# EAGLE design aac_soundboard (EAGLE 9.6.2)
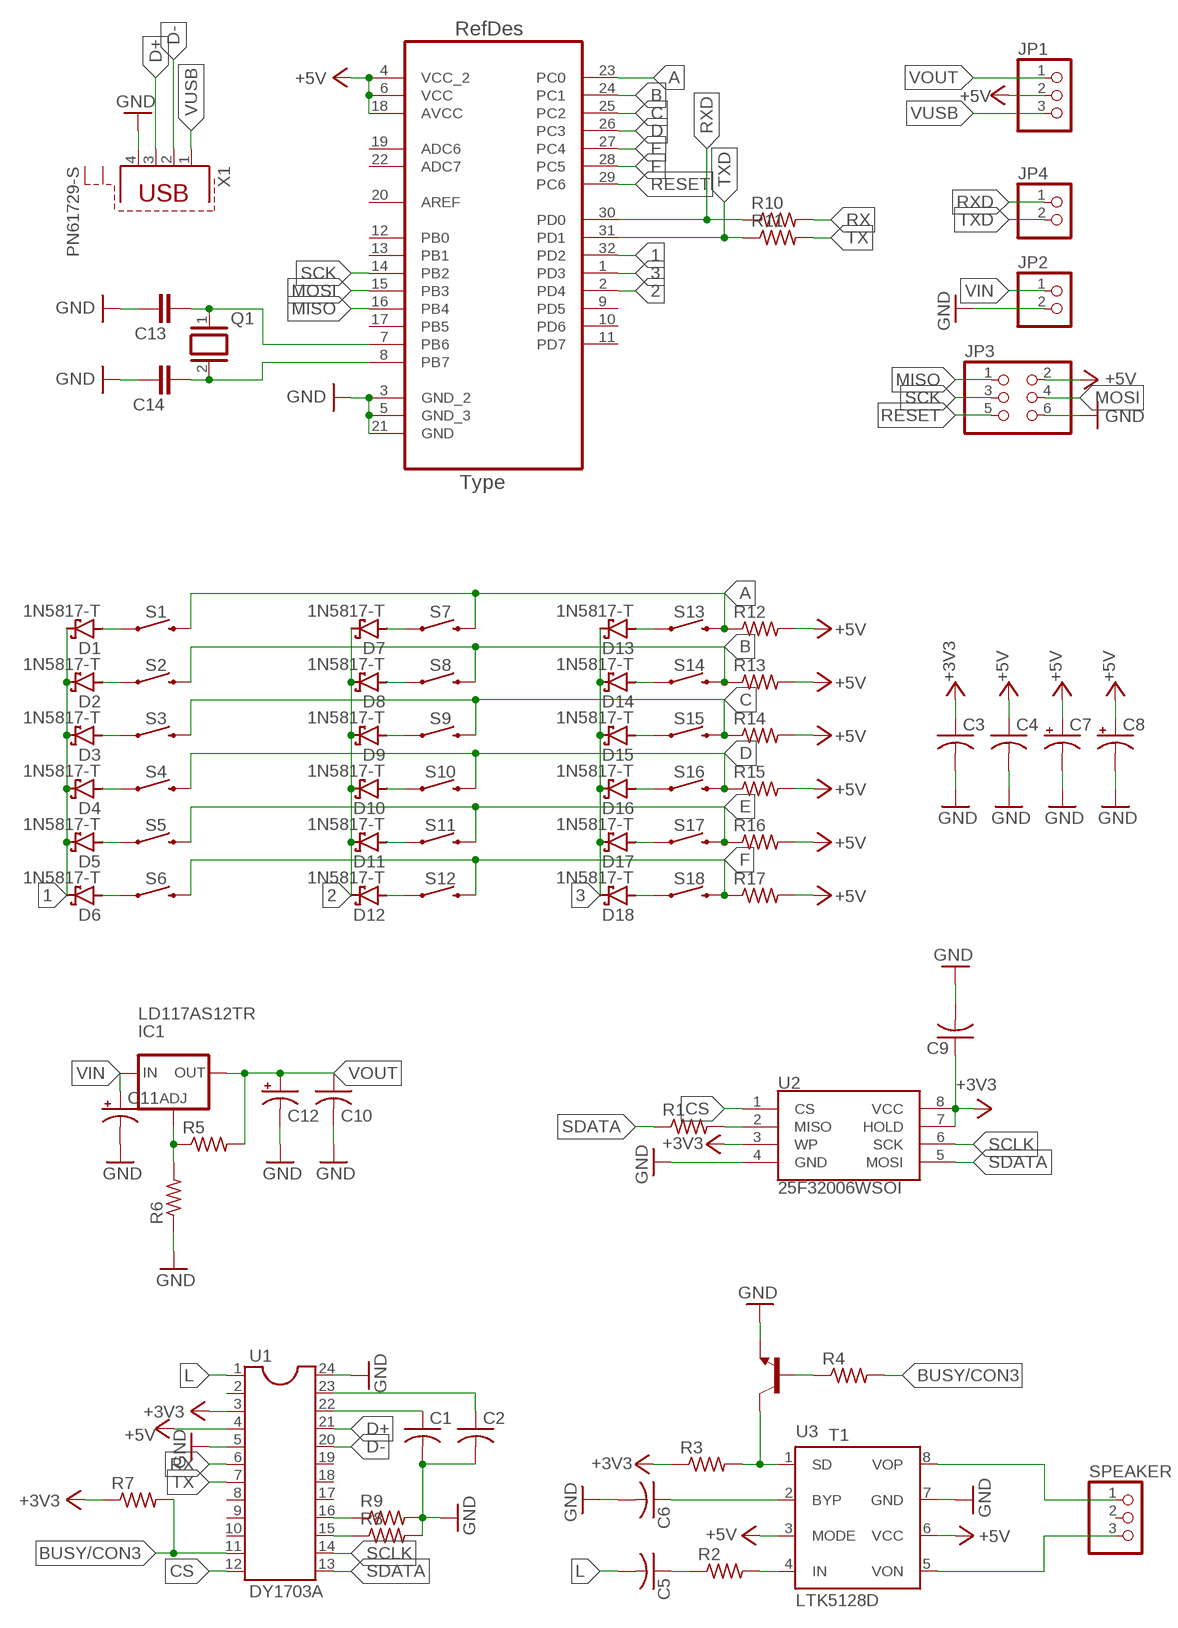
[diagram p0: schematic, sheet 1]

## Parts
ATMEGA328  ATMEGA328P-AU  [QFP80P900X900X120-32N]
C1  C-US050-025X075  [C050-025X075]
C2  C-US050-025X075  [C050-025X075]
C3  C-US050-025X075  [C050-025X075]
C4  C-US050-025X075  [C050-025X075]
C5  C-US050-025X075  [C050-025X075]
C6  C-US050-025X075  [C050-025X075]
C7  CPOL-USE2.5-6  [E2,5-6]
C8  CPOL-USE2.5-6  [E2,5-6]
C9  C-US050-025X075  [C050-025X075]
C10  C-US050-025X075  [C050-025X075]
C11  CPOL-USE2.5-6  [E2,5-6]
C12  CPOL-USE2.5-6  [E2,5-6]
C13  C-EU025-024X044  [C025-024X044]
C14  C-EU025-024X044  [C025-024X044]
D1  1N5817-T  [DO41-7.6]
D2  1N5817-T  [DO41-7.6]
D3  1N5817-T  [DO41-7.6]
D4  1N5817-T  [DO41-7.6]
D5  1N5817-T  [DO41-7.6]
D6  1N5817-T  [DO41-7.6]
D7  1N5817-T  [DO41-7.6]
D8  1N5817-T  [DO41-7.6]
D9  1N5817-T  [DO41-7.6]
D10  1N5817-T  [DO41-7.6]
D11  1N5817-T  [DO41-7.6]
D12  1N5817-T  [DO41-7.6]
D13  1N5817-T  [DO41-7.6]
D14  1N5817-T  [DO41-7.6]
D15  1N5817-T  [DO41-7.6]
D16  1N5817-T  [DO41-7.6]
D17  1N5817-T  [DO41-7.6]
D18  1N5817-T  [DO41-7.6]
IC1  LD117AS12TR  [SOT223]
JP1  PINHD-1X3  [1X03]
JP2  PINHD-1X2  [1X02]
JP3  PINHD-2X3  [2X03]
JP4  PINHD-1X2  [1X02]
Q1  XTAL/S  [QS]
R1  R-US_0204/7  [0204/7]
R2  R-US_0204/7  [0204/7]
R3  R-US_0204/7  [0204/7]
R4  R-US_0204/7  [0204/7]
R5  R-US_0204/7  [0204/7]
R6  R-US_0204/7  [0204/7]
R7  R-US_0204/7  [0204/7]
R8  R-US_0204/7  [0204/7]
R9  R-US_0204/7  [0204/7]
R10  R-US_0204/7  [0204/7]
R11  R-US_0204/7  [0204/7]
R12  R-US_0204/7  [0204/7]
R13  R-US_0204/7  [0204/7]
R14  R-US_0204/7  [0204/7]
R15  R-US_0204/7  [0204/7]
R16  R-US_0204/7  [0204/7]
R17  R-US_0204/7  [0204/7]
S1  MOMENTARY-SWITCH-SPST-PTH-12MM  [TACTILE_SWITCH_PTH_12MM]
S2  MOMENTARY-SWITCH-SPST-PTH-12MM  [TACTILE_SWITCH_PTH_12MM]
S3  MOMENTARY-SWITCH-SPST-PTH-12MM  [TACTILE_SWITCH_PTH_12MM]
S4  MOMENTARY-SWITCH-SPST-PTH-12MM  [TACTILE_SWITCH_PTH_12MM]
S5  MOMENTARY-SWITCH-SPST-PTH-12MM  [TACTILE_SWITCH_PTH_12MM]
S6  MOMENTARY-SWITCH-SPST-PTH-12MM  [TACTILE_SWITCH_PTH_12MM]
S7  MOMENTARY-SWITCH-SPST-PTH-12MM  [TACTILE_SWITCH_PTH_12MM]
S8  MOMENTARY-SWITCH-SPST-PTH-12MM  [TACTILE_SWITCH_PTH_12MM]
S9  MOMENTARY-SWITCH-SPST-PTH-12MM  [TACTILE_SWITCH_PTH_12MM]
S10  MOMENTARY-SWITCH-SPST-PTH-12MM  [TACTILE_SWITCH_PTH_12MM]
S11  MOMENTARY-SWITCH-SPST-PTH-12MM  [TACTILE_SWITCH_PTH_12MM]
S12  MOMENTARY-SWITCH-SPST-PTH-12MM  [TACTILE_SWITCH_PTH_12MM]
S13  MOMENTARY-SWITCH-SPST-PTH-12MM  [TACTILE_SWITCH_PTH_12MM]
S14  MOMENTARY-SWITCH-SPST-PTH-12MM  [TACTILE_SWITCH_PTH_12MM]
S15  MOMENTARY-SWITCH-SPST-PTH-12MM  [TACTILE_SWITCH_PTH_12MM]
S16  MOMENTARY-SWITCH-SPST-PTH-12MM  [TACTILE_SWITCH_PTH_12MM]
S17  MOMENTARY-SWITCH-SPST-PTH-12MM  [TACTILE_SWITCH_PTH_12MM]
S18  MOMENTARY-SWITCH-SPST-PTH-12MM  [TACTILE_SWITCH_PTH_12MM]
SPEAKER  PINHD-1X3  [1X03]
T1  -NPN-TO92-EBC  [TO92-EBC]
U1  DY1703A  [TSSOP24]
U2  25F32006WSOI  SPI_FLASH-X25XXSMD1  [SO08-EIAJ]
U3  LTK5128D  [SO08_PAD]
X1  PN61729-S  [PN61729-S]

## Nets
1: ATMEGA328.32(PD2) D1.C D2.C D3.C D4.C D5.C D6.C
2: ATMEGA328.2(PD4) D7.C D8.C D9.C D10.C D11.C D12.C
3: ATMEGA328.1(PD3) D13.C D14.C D15.C D16.C D17.C D18.C
+3V3: C3.1 C9.1 R3.1 R7.1 U1.3 U2.3(WP) U2.7(HOLD) U2.8(VCC)
+5V: ATMEGA328.4(VCC_2) ATMEGA328.6(VCC) ATMEGA328.18(AVCC) C4.1 C7.+ C8.+ JP1.2 JP3.2 R12.2 R13.2 R14.2 R15.2 R16.2 R17.2 U1.4 U3.3(MODE) U3.6(VCC)
A: ATMEGA328.23(PC0) R12.1 S1.3 S7.3 S13.3
B: ATMEGA328.24(PC1) R13.1 S2.3 S8.3 S14.3
BUSY/CON3: R4.2 R7.2 U1.11
C: ATMEGA328.25(PC2) R14.1 S3.3 S9.3 S15.3
CON1: R9.1 U1.16
CON2: R8.1 U1.15
CS: U1.12 U2.1(CS)
D: ATMEGA328.26(PC3) R15.1 S4.3 S10.3 S16.3
D+: U1.21 X1.3
D-: U1.20 X1.2
E: ATMEGA328.27(PC4) R16.1 S5.3 S11.3 S17.3
F: ATMEGA328.28(PC5) R17.1 S6.3 S12.3 S18.3
GND: ATMEGA328.3(GND_2) ATMEGA328.5(GND_3) ATMEGA328.21(GND) C1.2 C2.2 C3.2 C4.2 C6.2 C7.- C8.- C9.2 C10.2 C11.- C12.- C13.2 C14.2 JP2.2 JP3.6 R6.1 R8.2 R9.2 T1.E U1.5 U1.24 U2.4(GND) U3.7(GND) X1.4
L: C5.2 U1.1
MISO: ATMEGA328.16(PB4) JP3.1
MOSI: ATMEGA328.15(PB3) JP3.4
N$1: D1.A S1.1
N$2: D2.A S2.1
N$3: D3.A S3.1
N$4: D4.A S4.1
N$5: D5.A S5.1
N$6: D6.A S6.1
N$7: D7.A S7.1
N$8: D8.A S8.1
N$9: D9.A S9.1
N$10: D10.A S10.1
N$11: D11.A S11.1
N$12: D12.A S12.1
N$13: D13.A S13.1
N$14: D14.A S14.1
N$15: D15.A S15.1
N$16: D16.A S16.1
N$17: D17.A S17.1
N$18: D18.A S18.1
N$28: R1.2 U2.2(MISO)
N$29: R2.2 U3.4(IN)
N$30: C6.1 U3.2(BYP)
N$31: C5.1 R2.1
N$32: R3.2 T1.C U3.1(SD)
N$33: R4.1 T1.B
N$34: C1.1 U1.22
N$35: C2.1 U1.23
N$36: IC1.1(ADJ) R5.1 R6.2
N$37: SPEAKER.1 U3.8(VOP)
N$38: SPEAKER.3 U3.5(VON)
N$40: ATMEGA328.8(PB7) C14.1 Q1.2
N$41: ATMEGA328.7(PB6) C13.1 Q1.1
RESET: ATMEGA328.29(PC6) JP3.5
RX: R10.2 U1.6
RXD: ATMEGA328.30(PD0) JP4.1 R10.1
SCK: ATMEGA328.14(PB2) JP3.3
SCLK: U1.14 U2.6(SCK)
SDATA: R1.1 U1.13 U2.5(MOSI)
TX: R11.2 U1.7
TXD: ATMEGA328.31(PD1) JP4.2 R11.1
VIN: C11.+ IC1.3(IN) JP2.1
VOUT: C10.1 C12.+ IC1.4(OUT) JP1.1 R5.2
VUSB: JP1.3 X1.1
Unconnected: ATMEGA328.9(PD5) ATMEGA328.10(PD6) ATMEGA328.11(PD7) ATMEGA328.12(PB0) ATMEGA328.13(PB1) ATMEGA328.17(PB5) ATMEGA328.19(ADC6) ATMEGA328.20(AREF) ATMEGA328.22(ADC7) SPEAKER.2 U1.2 U1.8 U1.9 U1.10 U1.17 U1.18 U1.19 X1.S1 X1.S2

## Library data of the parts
ATMEGA328 = Atmel-ATMEGA328P-AU:ATMEGA328P-AU; DESCRIPTION: 8-bit Microcontroller with In-System Programmable Flash; MPN: ATMEGA328P-AU; OC_FARNELL: 1715486; OC_NEWARK: 14R4631; PACKAGE: TQFP-32; SUPPLIER: Atmel
C1-C6 C9 C10 = rcl:C-US: CAPACITOR, American symbol; SPICEPREFIX: C
C7 C8 C11 C12 = rcl:CPOL-US: POLARIZED CAPACITOR, American symbol; SPICEPREFIX: C
C13 C14 = rcl:C-EU: CAPACITOR, European symbol; SPICEPREFIX: C
D1-D18 = diode:1N581*: 1.0A SCHOTTKY BARRIER RECTIFIER
IC1 = v-reg:LD117A?*: Low drop fixed and adjustable positive voltage regulators 1 A Source: http://www.st.com/stonline/products/literature/ds/7194/ld1117axx.pdf
JP1 SPEAKER = pinhead:PINHD-1X3: PIN HEADER
JP2 JP4 = pinhead:PINHD-1X2: PIN HEADER
JP3 = pinhead:PINHD-2X3: PIN HEADER
Q1 = special:XTAL/S: CRYSTAL
R1-R17 = rcl:R-US_: RESISTOR, American symbol; SPICEPREFIX: R
S1-S18 = SparkFun-Switches:MOMENTARY-SWITCH-SPST: Momentary Switch (Pushbutton) - SPST; PROD_ID: SWCH-09185; SF_SKU: COM-09190
T1 = transistor:*-NPN-: NPN Transistror BF959 corrected 2008.03.06
U1 = smd_sop8_amp:DY1703A
U2 = SparkFun-IC-Memory:SPI_FLASH-X25XX: 32M Serial Flash Memory 8pin SPI Flash series x25xx. Works with devices like W25X32 and BR25L32 Datasheet SparkFun Products SparkFun Venus GPS Logger (GPS-10920); PROD_ID: IC-09109
U3 = smd_sop8_amp:LTK5128D
X1 = con-berg:PN61729-S: BERG USB connector; OC_FARNELL: unknown; OC_NEWARK: unknown

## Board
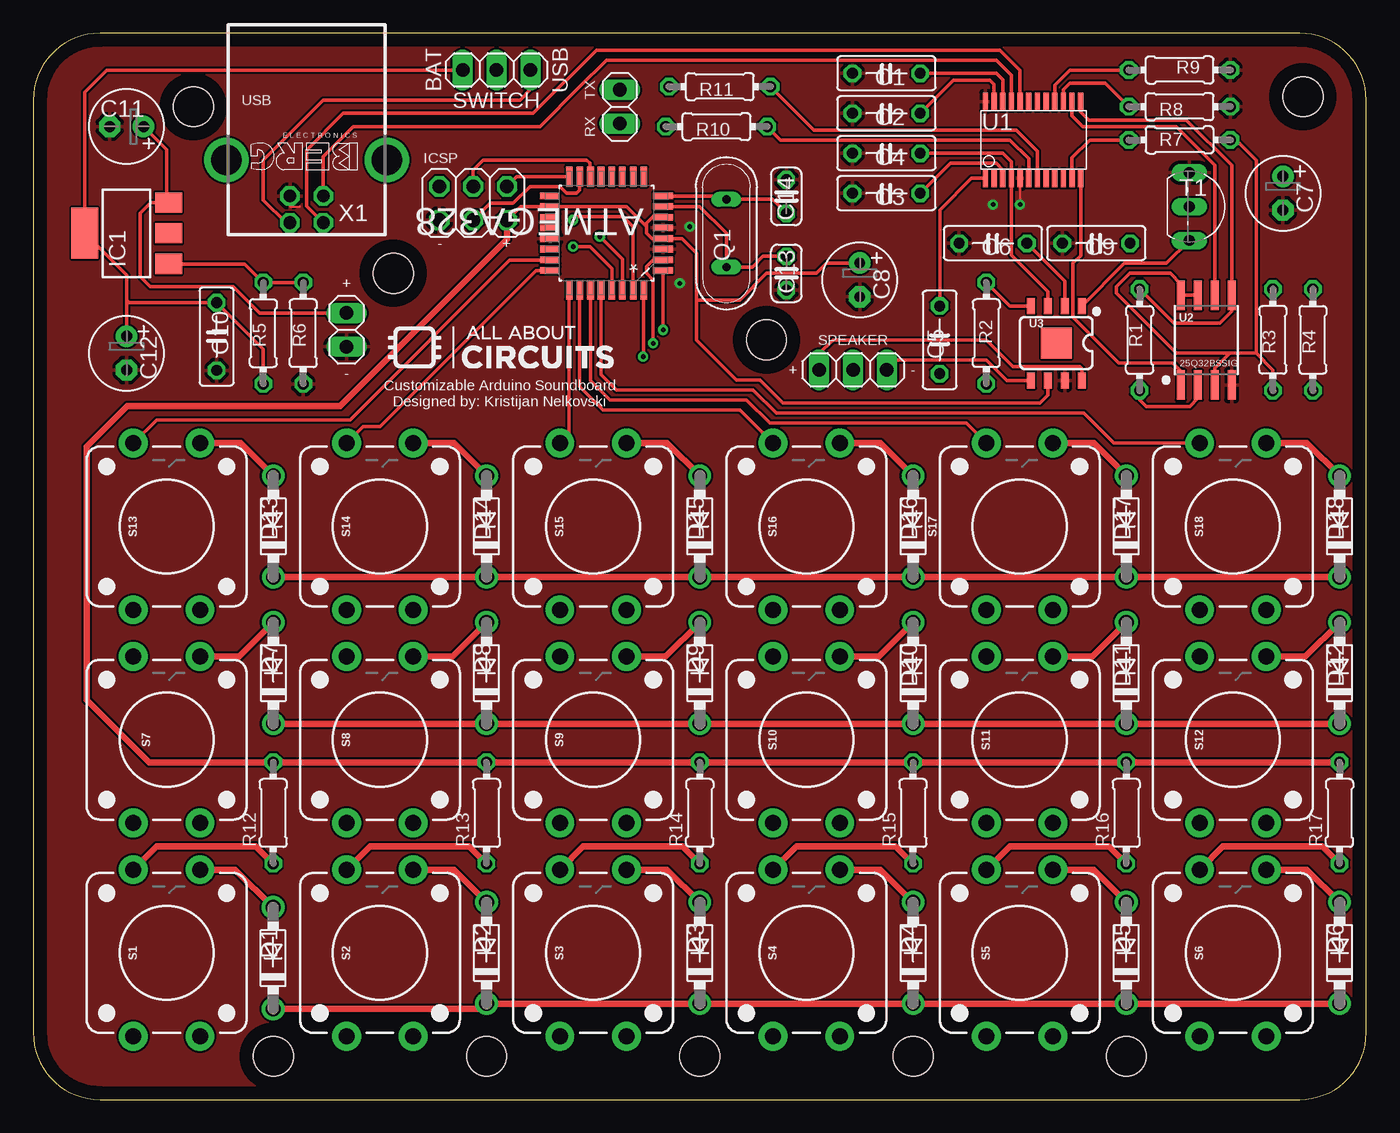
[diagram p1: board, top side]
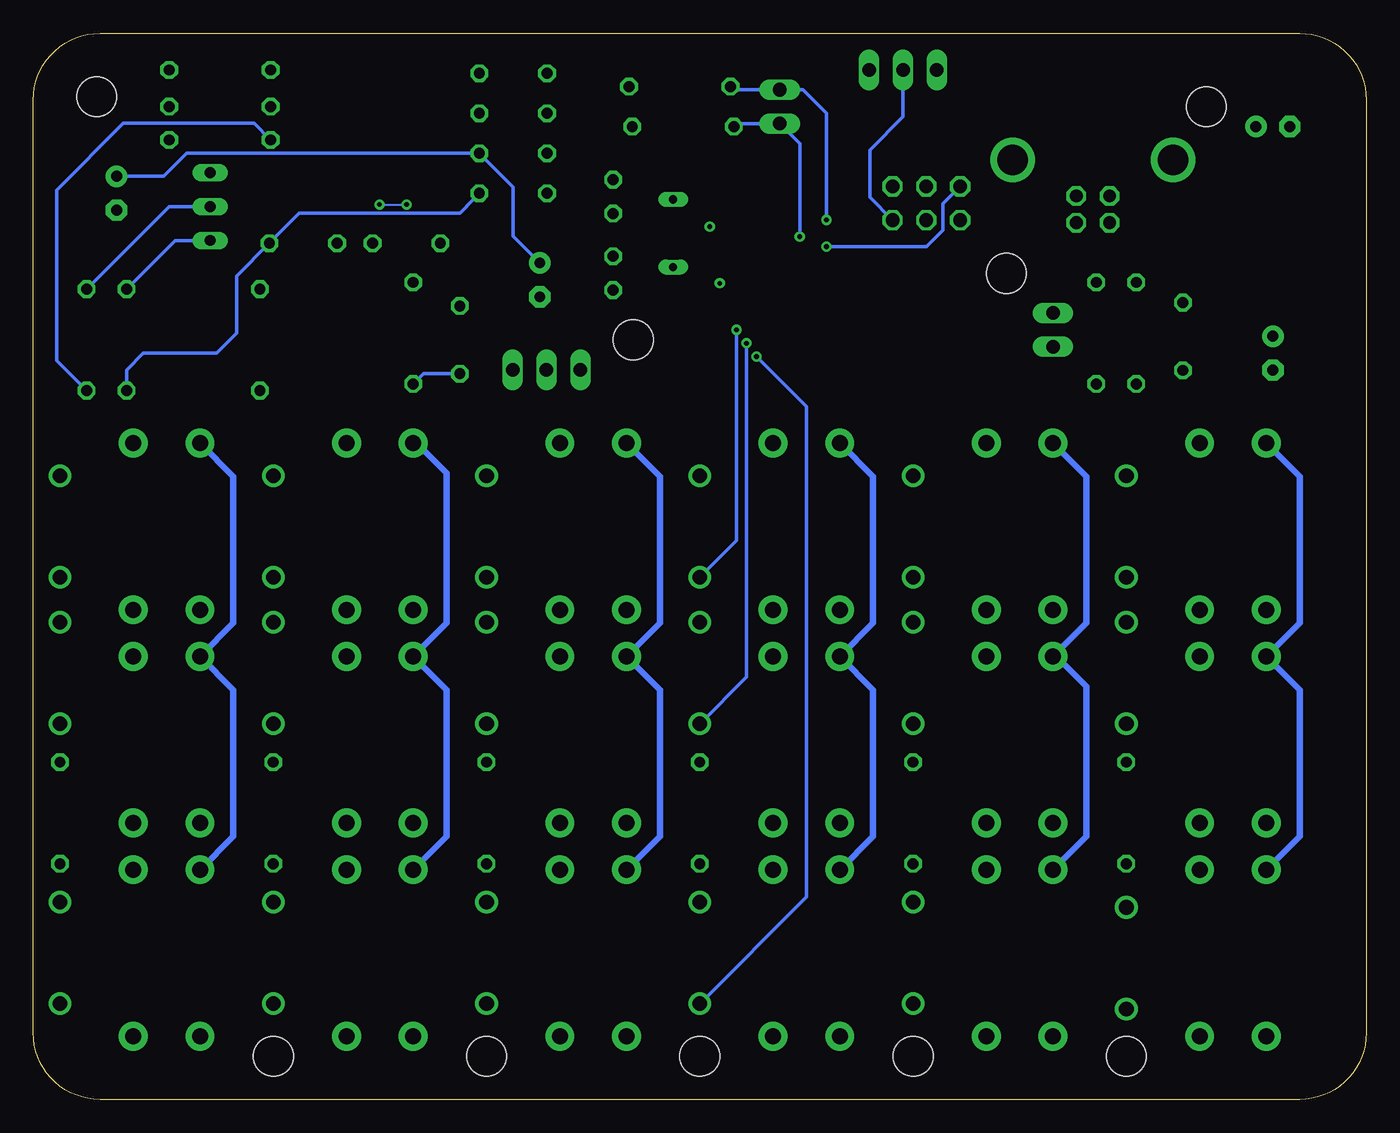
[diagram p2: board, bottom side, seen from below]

Size 100 x 80 mm. Coordinates in mm from the lower left corner, seen from the top.
Outline: 0,75 0,5 arc90 5,0 95,0 arc90 100,5 100,75 arc90 95,80 5,80 arc90 0,75
Copper layers (1*16): Top 0.035mm / dielectric 1.5mm / Bottom 0.035mm
Design rules "default": minimum track width 6mil, minimum drill 0.35mm, track to track 6mil, track to pad 6mil, pad to pad 6mil, via to via 6mil, smd to smd 6mil, copper to edge 40mil, drill to drill 6mil, minimum pad ring 10mil, minimum via ring 8mil, stop-mask expansion 4mil, vias tented up to drill 0mil, thermal gap 10mil
Holes 3 mm at 18,3.25 34,3.25 50,3.25 66,3.25 82,3.25 55,57 27,62 12,74.5 95.25,75.25

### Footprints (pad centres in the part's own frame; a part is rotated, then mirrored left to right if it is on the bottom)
QFP80P900X900X120-32N = smd 1.473 x 0.508: 1 -4.242,2.794; 2 -4.242,2.007; 3 -4.242,1.194; 4 -4.242,0.406; 5 -4.242,-0.406; 6 -4.242,-1.194; 7 -4.242,-2.007; 8 -4.242,-2.794; 17 4.242,-2.794; 18 4.242,-2.007; 19 4.242,-1.194; 20 4.242,-0.406; 21 4.242,0.406; 22 4.242,1.194; 23 4.242,2.007; 24 4.242,2.794 | smd 0.508 x 1.473: 9 -2.794,-4.242; 10 -2.007,-4.242; 11 -1.194,-4.242; 12 -0.406,-4.242; 13 0.406,-4.242; 14 1.194,-4.242; 15 2.007,-4.242; 16 2.794,-4.242; 25 2.794,4.242; 26 2.007,4.242; 27 1.194,4.242; 28 0.406,4.242; 29 -0.406,4.242; 30 -1.194,4.242; 31 -2.007,4.242; 32 -2.794,4.242
C050-025X075 = drill 0.813 octagon: 1 -2.54,0; 2 2.54,0
E2,5-6 = drill 0.813 pad 1.6: + -1.27,0 | drill 0.813 pad 1.6 octagon: - 1.27,0
C025-024X044 = drill 0.813 octagon: 1 -1.27,0; 2 1.27,0
DO41-7.6 = drill 1.1 pad 1.7: A 3.81,0; C -3.81,0
SOT223 = smd 1.5 x 2: 1 -2.3,-3.15; 2 0,-3.15; 3 2.3,-3.15 | smd 3.8 x 2: 4 0,3.15
1X03 = drill 1.016 long: 1 -2.54,0; 2 0,0; 3 2.54,0
1X02 = drill 1.016 long: 1 -1.27,0; 2 1.27,0
2X03 = drill 1.016 octagon: 1 -2.54,-1.27; 2 -2.54,1.27; 3 0,-1.27; 4 0,1.27; 5 2.54,-1.27; 6 2.54,1.27
QS = drill 0.61 long: 1 -2.54,0; 2 2.54,0
0204/7 = drill 0.813 octagon: 1 -3.81,0; 2 3.81,0
TACTILE_SWITCH_PTH_12MM = drill 1.2 pad 2.159: 1 6.25,-2.5; 2 -6.25,-2.5; 3 6.25,2.5; 4 -6.25,2.5
TO92-EBC = drill 0.813 long: B 0,-1.27; C 2.54,-1.27; E -2.54,-1.27
TSSOP24 = smd 0.4 x 1.35: 1 -3.575,-2.875; 2 -2.925,-2.875; 3 -2.275,-2.875; 4 -1.625,-2.875; 5 -0.975,-2.875; 6 -0.325,-2.875; 7 0.325,-2.875; 8 0.975,-2.875; 9 1.625,-2.875; 10 2.275,-2.875; 11 2.93,-2.872; 12 3.58,-2.872; 13 3.573,2.875; 14 2.923,2.875; 15 2.275,2.875; 16 1.625,2.875; 17 0.975,2.875; 18 0.325,2.875; 19 -0.325,2.875; 20 -0.975,2.875; 21 -1.625,2.875; 22 -2.275,2.875; 23 -2.925,2.875; 24 -3.575,2.875
SO08-EIAJ = smd 0.61 x 2.21: 1 -1.905,-3.378; 2 -0.635,-3.378; 3 0.635,-3.378; 4 1.905,-3.378; 5 1.905,3.353; 6 0.635,3.353; 7 -0.635,3.353; 8 -1.905,3.353
SO08_PAD = smd 0.6 x 1.2: 1 -1.905,-2.8; 2 -0.635,-2.8; 3 0.635,-2.8; 4 1.905,-2.8; 5 1.905,2.8; 6 0.635,2.8; 7 -0.635,2.8; 8 -1.905,2.8 | smd 2.311 x 2.311: PAD 0,0
PN61729-S = drill 0.95 octagon: 1 1.25,4.71; 2 -1.25,4.71; 3 -1.25,2.71; 4 1.25,2.71 | drill 2.3 pad 2.9: S1 -6.02,0; S2 6.02,0

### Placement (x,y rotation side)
ATMEGA328  43,65 180 top
C1  64,77 180 top
C2  64,74 180 top
C3  64,68 180 top
C4  64,71 180 top
C5  68,57 90 top
C6  72,64.25 180 top
C7  93.75,68 270 top
C8  62,61.5 270 top
C9  79.75,64.25 180 top
C10  13.75,57.25 270 top
C11  7,73 180 top
C12  7,56 270 top
C13  56.5,62 270 top
C14  56.5,67.75 90 top
D1  17.99,10.61 90 top
D2  34,11 90 top
D3  50,11 90 top
D4  66,11 90 top
D5  82,11 90 top
D6  98,11 90 top
D7  18,32 90 top
D8  34,32 90 top
D9  50,32 90 top
D10  66,32 90 top
D11  82,32 90 top
D12  98,32 90 top
D13  18,43 90 top
D14  34,43 90 top
D15  50,43 90 top
D16  66,43 90 top
D17  82,43 90 top
D18  98,43 90 top
IC1  7,65 90 top
JP1  34.75,77.25 0 top
JP2  23.5,57.75 270 top
JP3  33,67.25 180 top
JP4  44,74.5 90 top
Q1  52,65 90 top
R1  83,57 270 top
R2  71.5,57.5 90 top
R3  93,57 90 top
R4  96,57 270 top
R5  17.25,57.5 270 top
R6  20.25,57.5 90 top
R7  86,72 180 top
R8  86,74.5 0 top
R9  86,77.25 0 top
R10  51.25,73 0 top
R11  51.5,76 0 top
R12  18,21.5 90 top
R13  34,21.5 90 top
R14  50,21.5 90 top
R15  66,21.5 90 top
R16  82,21.5 90 top
R17  98,21.5 90 top
S1  10,11 90 top
S2  26,11 90 top
S3  42,11 90 top
S4  58,11 90 top
S5  74,11 90 top
S6  90,11 90 top
S7  10,27 90 top
S8  26,27 90 top
S9  42,27 90 top
S10  58,27 90 top
S11  74,27 90 top
S12  90,27 90 top
S13  10,43 90 top
S14  26,43 90 top
S15  42,43 90 top
S16  58,43 90 top
S17  74,43 90 top
S18  90,43 90 top
SPEAKER  61.5,54.75 0 top
T1  88,67 270 top
U1  75,72 0 top
U2  88,57 0 top
U3  76.75,56.75 180 top
X1  20.5,70.5 180 top

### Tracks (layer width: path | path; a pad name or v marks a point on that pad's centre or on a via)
1  (via drill 0.35)
  Top 0.254: v45.75,55.75 45.79,55.79 ATMEGA328.32
  Top 0.5: D1.C 33.61,6.8 D2.C D3.C D4.C D5.C D6.C
  Bottom 0.254: v45.75,55.75 42,52 42,15.19 D3.C
2  (via drill 0.35)
  Top 0.254: ATMEGA328.2 46.51,62.99 46.5,63 46,62.5 46,62 46.5,61.5 v46.5,56.75
  Top 0.5: D12.C D11.C D10.C D9.C D8.C D7.C
  Bottom 0.254: v46.5,56.75 46.5,31.69 D9.C
3  (via drill 0.35)
  Top 0.152: D17.C 81.81,39.19
  Top 0.254: ATMEGA328.1 47.25,62.2 v47.25,57.75
  Top 0.5: D13.C D14.C D15.C D16.C 81.81,39.19 | D17.C D18.C
  Bottom 0.254: D15.C 47.25,41.94 v47.25,57.75
+3V3
  Top 0.254: U2.7 U2.8 86.09,61.2 85.29,62 82.25,62 81.25,61 81.25,60.5 85.75,56 89.75,56 | C3.1 68.79,70.25 72.25,70.25 72.75,69.75 72.75,69.15 U1.3 | U2.3 88.64,54.88 89.75,56 | 89.75,56 90.25,56 91.75,56 | 91.75,56 93,54.75 R3.1 | 91.75,56 91.75,70.5 90.25,72 R7.1
  Bottom 0.254: R3.1 93,54.75 91.75,56 86.25,56 84.75,57.5 84.75,61.79 C9.1 80.04,66.5 68,66.5 67.5,67 67.5,67.04 C3.1
+5V
  Top 0.254: JP3.2 36.57,67.01 ATMEGA328.18 44.49,67.01 46,65.5 | C4.1 72.75,71 73.38,70.38 U1.4 73.38,63.38 76.11,60.63 U3.3 | 46,65.5 46,65 46.41,64.59 ATMEGA328.4 48.66,64.59 49.75,63.5 49.75,60 | 46,65.5 46,65.75 46.5,66.25 47.19,66.25 ATMEGA328.6 | U3.6 76.11,52.87 75.5,52.25 56.25,52.25 54.5,54 52.75,54 49.75,57 49.75,60 | C8.+ 59.52,62.77 58.75,62 55,62 53,60 49.75,60
  Top 0.5: R17.2 R16.2 R15.2 R14.2 R13.2 R12.2 8.69,25.31 4,30 4,49 7.03,52.03 23,52.03 35.54,64.57 JP3.2
  Bottom 0.254: JP3.2 37.25,67.69 37.25,71.25 34.75,73.75 JP1.2 | C7.+ 90.23,69.27 88.5,71 C4.1 64,68.46 64,64.77 C8.+
A
  Top 0.254: ATMEGA328.23 35.74,62.99 23.75,51 9.25,51 S13.3
  Top 0.5: S1.3 9.25,19 16.69,19 R12.1
  Bottom 0.5: S13.3 5,46.75 5,35.75 S7.3 5,30.75 5,19.75 S1.3
B
  Top 0.254: ATMEGA328.24 37.71,62.21 26,50.5 24.75,50.5 S14.3
  Top 0.5: S2.3 25.25,19 32.69,19 R13.1
  Bottom 0.5: S2.3 21,19.75 21,31 23.25,33.25 S8.3 21,35.75 21,46.75 S14.3
BUSY/CON3
  Top 0.254: U1.11 77.93,70.68 79.25,72 R7.2
  Bottom 0.254: R7.2 83.44,73.25 93.25,73.25 98.25,68.25 98.25,55.44 R4.2
C
  Top 0.254: ATMEGA328.25 40.21,49.96 S15.3
  Top 0.5: S3.3 41.25,19 48.69,19 R14.1
  Bottom 0.5: S3.3 37,19.75 37,30.75 S9.3 37,35.75 37,46.75 S15.3
CON1
  Top 0.254: U1.16 76.62,76.12 77.75,77.25 R9.1
CON2
  Top 0.254: U1.15 77.28,75.78 77.75,76.25 80.44,76.25 R8.1
CS
  Top 0.254: U1.12 78.58,63.33 78,62.75 78,58.71 81.46,55.25 85.5,55.25 86.09,54.66 U2.1
D
  Top 0.254: ATMEGA328.26 40.99,53.51 42.75,51.75 53,51.75 S16.3
  Top 0.5: S4.3 57.25,19 64.69,19 R15.1
  Bottom 0.5: S4.3 53,19.75 53,30.75 S10.3 53,35.75 53,46.75 S16.3
D+
  Top 0.254: U1.21 73.38,76.88 72.25,78 42.99,78 40.95,75.95 38,73 24,73 21.75,70.75 X1.3
D-
  Top 0.254: U1.20 74.03,77.22 72.5,78.75 42.25,78.75 37.5,74 23.25,74 20.5,71.25 20.5,67.04 X1.2
E
  Top 0.254: ATMEGA328.27 41.81,53.94 43.25,52.5 53.5,52.5 55.25,50.75 70,50.75 S17.3
  Top 0.5: S5.3 73.25,19 80.69,19 R16.1
  Bottom 0.5: S5.3 69,19.75 69,30.75 S11.3 69,35.75 69,47 71.25,49.25 S17.3
F
  Top 0.254: ATMEGA328.28 42.59,54.41 43.75,53.25 54,53.25 55.75,51.5 78.8,51.5 81.05,49.25 S18.3
  Top 0.5: S6.3 89.25,19 96.69,19 R17.1
  Bottom 0.5: S6.3 85,19.75 85,30.75 S12.3 85,35.75 85,46.75 S18.3
GND  (via drill 0.35)
  Top 0.152: X1.4 19.25,67 20,67 | U1.5 v74.03,67.16
  Bottom 0.152: v74.03,67.16 v72,67.16
  other vias: 49.25,65.5 48.5,61.25
  pour Top: 0,0 0,80 1,80 100,80 100,0
L
  Top 0.254: C5.2 68,66.75 70.38,69.12 U1.1
MISO
  Top 0.254: ATMEGA328.16 36.26,69.24 JP3.1
MOSI
  Top 0.254: JP3.4 34.27,67.25 36,67.25 37.25,68.5 39.5,68.5 40,68 40.75,68 40.99,68.24 ATMEGA328.15
N$1
  Top 0.5: S1.1 15.16,17.25 D1.A
N$2
  Top 0.5: S2.1 31.56,17.25 D2.A
N$3
  Top 0.5: S3.1 47.56,17.25 D3.A
N$4
  Top 0.5: S4.1 63.56,17.25 D4.A
N$5
  Top 0.5: S5.1 79.56,17.25 D5.A
N$6
  Top 0.5: S6.1 95.56,17.25 D6.A
N$7
  Top 0.5: S7.1 15.44,33.25 D7.A
N$8
  Top 0.5: S8.1 31.44,33.25 D8.A
N$9
  Top 0.5: S9.1 47.44,33.25 D9.A
N$10
  Top 0.5: S10.1 63.44,33.25 D10.A
N$11
  Top 0.5: S11.1 79.44,33.25 D11.A
N$12
  Top 0.5: S12.1 95.44,33.25 D12.A
N$13
  Top 0.5: S13.1 15.56,49.25 D13.A
N$14
  Top 0.5: S14.1 31.56,49.25 D14.A
N$15
  Top 0.5: S15.1 47.56,49.25 D15.A
N$16
  Top 0.5: S16.1 63.56,49.25 D16.A
N$17
  Top 0.5: S17.1 79.56,49.25 D17.A
N$18
  Top 0.5: S18.1 95.56,49.25 D18.A
N$28
  Top 0.254: U2.2 87.36,52.62 86.75,52 83.5,52 83,52.5 R1.2
N$29
  Top 0.254: U3.4 73.26,59.55 R2.2
N$30
  Top 0.254: C6.1 77.39,61.41 U3.2
N$31
  Bottom 0.254: C5.1 70.73,54.46 R2.1
N$32
  Top 0.254: U3.1 81.86,62.75 85.02,62.75 T1.C
  Bottom 0.254: T1.C 89.35,64.46 R3.2
N$33
  Bottom 0.254: T1.B 89.81,67 R4.1
N$34
  Top 0.254: U1.22 72.72,76.53 72.25,77 C1.1
N$35
  Top 0.254: U1.23 72.08,76.17 71.75,76.5 69.04,76.5 C2.1
N$36
  Top 0.254: IC1.1 15.86,62.7 R5.1 R6.2
N$37
  Top 0.254: U3.8 78.66,54.84 78.5,55 73.5,55 71.5,57 60,57 58.96,55.96 SPEAKER.1
N$38
  Top 0.254: SPEAKER.3 64.79,55.5 71.5,55.5 73.05,53.95 U3.5
N$40
  Top 0.254: ATMEGA328.8 51.75,67.79 Q1.2 55.44,67.54 C14.1
N$41
  Top 0.254: ATMEGA328.7 49.99,67.01 52,65 Q1.1 53.94,62.46 54.75,63.27 C13.1
RESET  (via drill 0.35)
  Top 0.254: v40.5,64 41.75,64 43.41,62.34 ATMEGA328.29
  Bottom 0.254: JP3.5 31.75,67.23 31.75,65.25 33,64 v40.5,64
RX
  Top 0.254: U1.6 74.67,70.58 73.25,72 56.06,72 R10.2
RXD  (via drill 0.35)
  Top 0.254: v42.5,64.75 44.19,63.06 ATMEGA328.30
  Bottom 0.254: R10.1 47.21,73.23 JP4.1 42.5,71.73 v42.5,64.75
SCK
  Top 0.254: ATMEGA328.14 41.75,69.3 41.75,70.25 41.5,70.5 33.75,70.5 33,69.75 JP3.3
SCLK
  Top 0.254: U1.14 77.92,73.83 78.75,73 85.75,73 88.64,70.11 U2.6
SDATA
  Top 0.254: U1.13 78.57,74.12 79.2,73.5 86.5,73.5 89.91,70.09 U2.5 89.91,59.16 89,58.25 85.56,58.25 R1.1
TX
  Top 0.254: U1.7 75.33,71.17 73.75,72.75 73.25,72.75 73,72.75 58.56,72.75 R11.2
TXD  (via drill 0.35)
  Top 0.254: v40.5,66 40.75,66.25 44.25,66.25 45.01,65.49 ATMEGA328.31
  Bottom 0.254: R11.1 47.46,75.77 JP4.2 42.27,75.77 40.5,74 v40.5,66
VIN
  Top 0.254: JP2.1 16.98,59.02 15,61 8.75,61 8,61.75 8,66.5 8.8,67.3 10,67.3 | IC1.3 10,67.3 | C11.+ 10,71.27 10,67.3
VOUT
  Top 0.254: C12.+ 7,60 | 7,60 7,61.85 IC1.4 3.85,75.6 5.5,77.25 JP1.1 | 7,60 7.21,59.79 C10.1 17.25,56.29 R5.2
VUSB
  Top 0.254: JP1.3 37.29,75.79 36.5,75 21.75,75 17.25,70.5 17.25,67.5 18.96,65.79 X1.1

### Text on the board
tPlace: BAT | USB | TX | USB | SWITCH | RX | ICSP | - | + | + | SPEAKER | + | - | 25Q32BSSIG | - | Customizable Arduino Soundboard / Designed by: Kristijan Nelkovski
